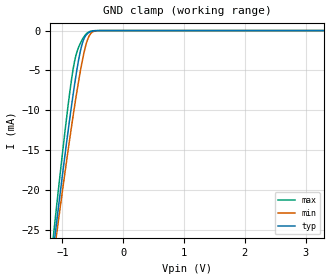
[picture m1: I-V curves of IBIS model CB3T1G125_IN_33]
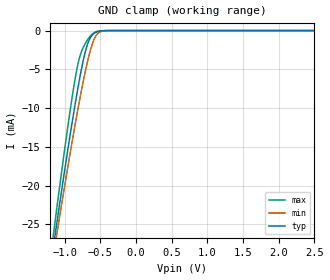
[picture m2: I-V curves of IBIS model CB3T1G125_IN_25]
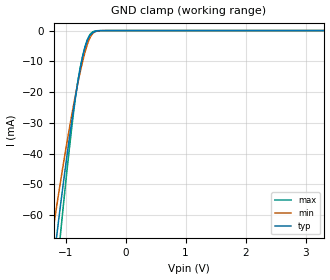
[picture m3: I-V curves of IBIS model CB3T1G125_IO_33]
| TEXAS INSTRUMENTS INCORPORATED
| Standard Linear and Logic Group
| IBIS Model of SN74CB3T1G125
| 3.3V LOW VOLTAGE SINGLE FET BUS SWITCH WITH 5V TOLERANT/LEVEL SHIFTER
| This file contains package information for the following:
|  SOT 5-pin (DBV) package as [Component] CB3T1G125_DBV
|  SOT 5-pin (DCK) package as [Component] CB3T1G125_DCK
| This device can be powered at the following Vccs:
|  3.3 volt Vcc
|  2.5 volt Vcc
| This file provides unique models under the [Model Selector] for each Vcc.
| For operation at a specific Vcc, select the appropriate model after each
| [Model Selector] keyword.
[IBIS Ver]   3.2
[Comment char]  |_char
[File Name]   sn74cb3t1g125.ibs
[File Rev]   1.1 | x_die
[Date]   August 1, 2003
[Source]   Data created from TI-SPICE simulations at TI-SLL.
[Notes]   The following is an IBIS list for the CB3T1G125.
   Please contact sllibis@ti.com with questions and
   comments concerning SLL IBIS models.
   - Non-monotonic data due to FET characteristics.
   - Power-clamp data has been deleted since there is no
   power-clamp diode in the device.
[Disclaimer] Property of Texas Instruments Incorporated.  Unauthorized
   reproduction and/or distribution is strictly prohibited.
   This product is protected under copyright law.
   Created  2003, (C) Copyright  2003, Texas Instruments
   Incorporated, All Rights Reserved
   UNLESS THERE IS A SIGNED, WRITTEN AGREEMENT TO THE
   CONTRARY, TEXAS INSTRUMENTS (TI) IS PROVIDING THE IBIS
   MODELS  AND WITHOUT ANY WARRANTY, EXPRESSED OR
   IMPLIED.  TI assumes no liability for:
   1) the accuracy of the IBIS models provided to your
   company;
   2) the proper functioning of these IBIS Models in your
   design or for any resulting applications; or
   3) infringement of patents, copyrights or intellectual
   property rights resulting from your use of these IBIS
   models.
   TI provides IBIS Models as a service to our customers.
   You and your company shall not distribute, sell or give
   these models to anyone else without prior written
   permission from TI.
   TI reserves the right to make changes to our products or
   to discontinue any semiconductor product or service
   without notice, and advises our customers to obtain the
   latest version of relevant information to verify, before
   placing orders, that the information being relied on is
   current.
   Please be aware that your receipt and use of the IBIS
   information provided shall serve as acceptance of these
   terms and conditions.  If you do not accept these terms,
   you should return or destroy the IBIS models and any
   other accompanying information immediately.
| Component CB3T1G125_DBV 5-pin SOT
[Component]   CB3T1G125_DBV
[Manufacturer]   Texas Instruments, Inc.
[Package]
|   typ   min   max
R_pkg   2.500e-02   2.100e-02   2.900e-02
L_pkg   1.529e-09   1.312e-09   1.906e-09
C_pkg   1.560e-13   1.100e-13   2.400e-13
[Pin]   signal_name   model_name   R_pin   L_pin   C_pin
1   NOE   CB3T1G125_IN   2.100e-02   1.511e-09   1.440e-13
2   A   CB3T1G125_IO   2.300e-02   1.312e-09   1.380e-13
3   GND   GND   2.900e-02   1.906e-09   2.400e-13
4   B   CB3T1G125_IO   2.600e-02   1.541e-09   1.500e-13
5   VCC   POWER   2.500e-02   1.374e-09   1.100e-13
| Component CB3T1G125_DCK 5-pin SOT
[Component]   CB3T1G125_DCK
[Manufacturer]   Texas Instruments, Inc.
[Package]
|   typ   min   max
R_pkg   2.000e-02   1.700e-02   2.500e-02
L_pkg   0.998e-09   0.881e-09   1.069e-09
C_pkg   1.460e-13   1.180e-13   2.050e-13
[Pin]   signal_name   model_name   R_pin   L_pin   C_pin
1   NOE   CB3T1G125_IN   1.900e-02   1.069e-09   1.620e-13
2   A   CB3T1G125_IO   1.800e-02   0.881e-09   1.210e-13
3   GND   GND   1.700e-02   1.031e-09   2.050e-13
4   B   CB3T1G125_IO   2.000e-02   0.960e-09   1.240e-13
5   VCC   POWER   2.500e-02   1.049e-09   1.180e-13
[Series Switch Groups]
| Function Group States
On  1 /   | A->B NOE,LOW
Off 1 /   | NOE,HIGH disable
[Series Pin Mapping]   pin_2   model_name   function_table_group
2   4   CB3T1G125_IO_33_S   1
| 2   4   CB3T1G125_IO_25_S   1
| Model CB3T1G125_IN
[Model Selector]   CB3T1G125_IN
CB3T1G125_IN_33   3.3 volt Vcc
CB3T1G125_IN_25   2.5 volt Vcc
| Model CB3T1G125_IO
[Model Selector]   CB3T1G125_IO
CB3T1G125_IO_33   3.3 volt Vcc
CB3T1G125_IO_25   2.5 volt Vcc
| Model CB3T1G125_IO_S
[Model Selector]   CB3T1G125_IO_S
CB3T1G125_IO_33_S   3.3 volt Vcc
CB3T1G125_IO_25_S   2.5 volt Vcc
[Model]   CB3T1G125_IO_33_S
Model_type  Series_switch
| variable   typ   min   max
C_comp   0   0   0
[Temperature Range]   40   100   -40
| Ambient temperature   25   85   -40
[Voltage range]   3.3   3   3.6
[On]
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[Off]
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[Model]   CB3T1G125_IO_25_S
Model_type  Series_switch
| variable   typ   min   max
C_comp   0   0   0
[Temperature Range]   40   100   -40
| Ambient temperature   25   85   -40
[Voltage range]   2.5   2.3   2.7
[On]
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[Off]
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| Models and submodels in the file (6): CB3T1G125_IN_33 (Input), CB3T1G125_IN_25 (Input), CB3T1G125_IO_33_S (Series_switch), CB3T1G125_IO_33 (Terminator), CB3T1G125_IO_25_S (Series_switch), CB3T1G125_IO_25 (Terminator)
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[Model]   CB3T1G125_IN_33
Model_type  Input
Vinl=0.8
Vinh=2.0
| variable   typ   min   max
C_comp   2.33pF   1.78pF   2.98pF
[Temperature Range]   40   100   -40
| Ambient temperature   25   85   -40
[Voltage range]   3.3   3   3.6
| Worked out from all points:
|   GND clamp passes 1 mA (typ) near -0.64 V on its own axis
[GND Clamp]
| CB3T1G125_IN_33
|   Voltage   I(typ)   I(min)   I(max)
-5.5V     -338.9mA   -314.3mA   -369mA
-1.14V    -26.82mA   -28.07mA   -25.13mA
-1.105V   -24.61mA   -26.05mA   -22.65mA
-1.075V   -22.73mA   -24.34mA   -20.55mA
-915mV    -13.07mA   -15.45mA   -9.893mA
-860mV    -9.954mA   -12.53mA   -6.658mA
-805mV    -7.019mA   -9.733mA   -4.027mA
-730mV    -3.528mA   -6.174mA   -2.02mA
-665mV    -1.428mA   -3.486mA   -1.009mA
-585mV    -362.1uA   -1.111mA   -263.9uA
-510mV    -78.77uA   -204.1uA   -38.82uA
3.3V      76.2pA     212.8pA    43.07pA
[Model]   CB3T1G125_IN_25
Model_type  Input
Vinl=0.7
Vinh=1.7
| variable   typ   min   max
C_comp   2.39pF   1.89pF   2.97pF
[Temperature Range]   40   100   -40
| Ambient temperature   25   85   -40
[Voltage range]   2.5   2.3   2.7
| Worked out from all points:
|   GND clamp passes 1 mA (typ) near -0.64 V on its own axis
[GND Clamp]
| CB3T1G125_IN_25
|   Voltage   I(typ)   I(min)   I(max)
-5.5V     -338.9mA   -314.3mA   -369mA
-1.17V    -28.73mA   -29.82mA   -27.27mA
-1.13V    -26.19mA   -27.5mA    -24.42mA
-1.095V   -23.98mA   -25.48mA   -21.95mA
-925mV    -13.65mA   -15.98mA   -10.52mA
-825mV    -8.06mA    -10.74mA   -4.88mA
-775mV    -5.531mA   -8.266mA   -3.027mA
-700mV    -2.416mA   -4.874mA   -1.51mA
-590mV    -396.4uA   -1.217mA   -293.2uA
-515mV    -88.16uA   -231.8uA   -44.89uA
-395mV    -4.232uA   -9.445uA   -775nA
2.5V      57.25pA    176.8pA    32.61pA
[Model]   CB3T1G125_IO_33
Model_type  Terminator
| variable   typ   min   max
C_comp   3.99pF   3.07pF   5.16pF
| C_tri-state   3.99pF   3.07pF   5.16pF
[Temperature Range]   40   100   -40
| Ambient temperature   25   85   -40
[Voltage range]   3.3   3   3.6
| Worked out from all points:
|   GND clamp passes 1 mA (typ) near -0.57 V on its own axis
[GND Clamp]
| CB3T1G125_IO_33
|   Voltage   I(typ)   I(min)   I(max)
-5.5V     -966.8mA   -814.4mA   -1.126A
-1.24V    -81.94mA   -69.05mA   -97.97mA
-1.195V   -74.51mA   -63.17mA   -88.59mA
-1.15V    -67.23mA   -57.4mA    -79.37mA
-1.11V    -60.89mA   -52.38mA   -71.31mA
-1.07V    -54.68mA   -47.46mA   -63.4mA
-905mV    -30.71mA   -28.4mA    -32.96mA
-785mV    -15.64mA   -16.16mA   -15.28mA
-675mV    -5.395mA   -6.944mA   -5.257mA
-565mV    -988.9uA   -1.385mA   -696.1uA
-415mV    -29.05uA   -40.98uA   -6.583uA
3.3V      246.5pA    10.98nA    81.94pA
